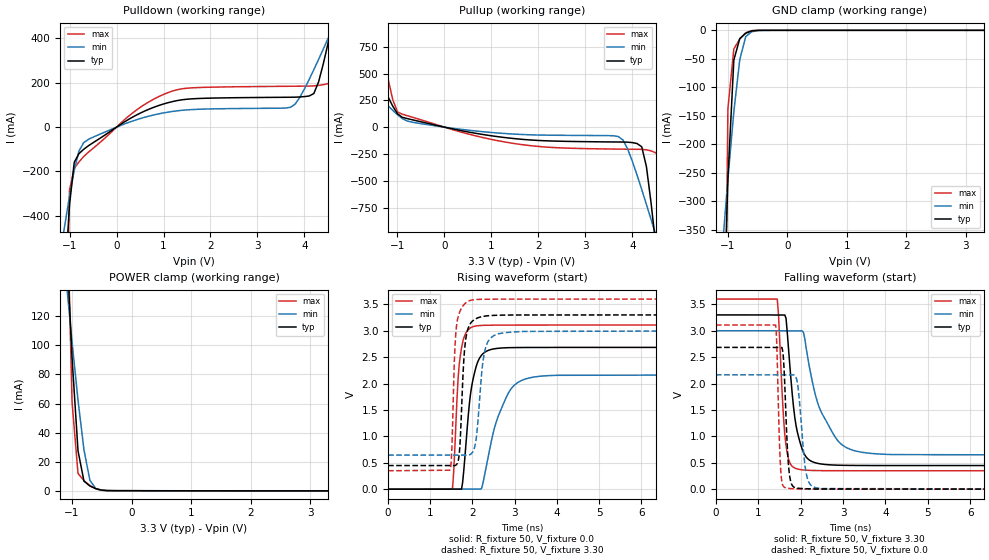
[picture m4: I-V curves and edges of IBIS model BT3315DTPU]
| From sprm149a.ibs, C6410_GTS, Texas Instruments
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[Model]   BT3315DTPU
Model_type   I/O
Vinh = 2.00
Vinl = 0.80
Enable   Active-Low
Polarity   Non-Inverting
| signals   A, GZ, Y
Vmeas = 1.5
|   typ   min   max
C_comp   1.6130p   1.5354p   1.7989p
|   typ   min   max
[Temperature Range]   25   -40   125
|   typ   min   max
[Voltage Range]   3.30V   3.00V   3.60V
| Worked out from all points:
|   slope of the pulldown table from 0 to 0.495 V, typ, clamps not added: 7.97 ohm
|   slope of the pullup table from 0 to 0.495 V, typ, clamps not added: 11.2 ohm
|   GND clamp passes 1 mA (typ) near -0.60 V on its own axis
|   POWER clamp passes 1 mA (typ) near -0.56 V on its own axis
|   rising waveform, R_fixture 50, V_fixture 0.0: 20-80 % time 219ps typ, 469ps min, 133ps max; typ from 0 V to 2.69 V
|   falling waveform, R_fixture 50, V_fixture 3.30: 20-80 % time 235ps typ, 561ps min, 133ps max; typ from 3.3 V to 0.447 V
|   rising waveform, R_fixture 50, V_fixture 3.30: 20-80 % time 109ps typ, 160ps min, 84.2ps max; typ from 0.447 V to 3.3 V
|   falling waveform, R_fixture 50, V_fixture 0.0: 20-80 % time 89.3ps typ, 141ps min, 67.2ps max; typ from 2.69 V to 0 V
[Pulldown]
|   Voltage   I(typ)   I(min)   I(max)
-3.3V     -10.57A    -3.704A    -44.33A
-1.1V     -692.7mA   -440.2mA   -1.224A
-1V       -348.9mA   -310.5mA   -283mA
-900mV    -158.9mA   -194.3mA   -185.9mA
-700mV    -100.1mA   -70.14mA   -132.7mA
1V        104.5mA    64.15mA    147.5mA
3.7V      134.9mA    89.32mA    184.4mA
4.2V      151.5mA    259.2mA    186.2mA
4.6V      471.8mA    446.1mA    223mA
4.7V      570.7mA    493.9mA    367.4mA
4.8V      671.3mA    542mA      570.8mA
6.6V      2.552A     1.425A     4.922A
[GND_clamp]
|   Voltage   I(typ)   I(min)   I(max)
-3.3V     -10.46A    -3.63A     -44.21A
-1.1V     -613.5mA   -391.3mA   -1.123A
-1V       -261.1mA   -261.1mA   -137.8mA
-900mV    -52.05mA   -142.6mA   -32.57mA
-800mV    -14.47mA   -51.16mA   -15.18mA
-700mV    -5.111mA   -10.97mA   -4.271mA
-600mV    -965.9uA   -2.449mA   -468.2uA
-400mV    -4.855uA   -52.49uA   -479.3nA
3.3V      88.82pA    4.205uA    44.41pA
[Pullup]
|   Voltage   I(typ)   I(min)   I(max)
-3.3V     2.442A     1.205A     5.525A
-2.7V     1.813A     912.6mA    4.046A
-1.9V     980.9mA    525.9mA    2.088A
-1.5V     573.5mA    336.5mA    1.13A
-1.1V     195.3mA    156.4mA    256.1mA
-800mV    80.54mA    58.25mA    108mA
3.7V      -138.7mA   -87.82mA   -205mA
4.2V      -183.2mA   -582.4mA   -207.6mA
4.5V      -1.109A    -1.007A    -239.2mA
4.6V      -1.528A    -1.151A    -325.8mA
4.7V      -1.958A    -1.297A    -1.261A
6.6V      -10.56A    -4.136A    -38.31A
[POWER_clamp]
|   Voltage   I(typ)   I(min)   I(max)
-3.3V     2.438A     1.199A     5.524A
-1.1V     176.6mA    145.4mA    226.9mA
-1V       91.69mA    102.4mA    60.94mA
-900mV    27.5mA     62.33mA    11.91mA
-800mV    6.572mA    28.18mA    6.905mA
-700mV    3.22mA     7.14mA     3.606mA
-600mV    1.379mA    1.452mA    1.304mA
-500mV    357.9uA    341.4uA    241uA
-400mV    65.66uA    67.61uA    56.94uA
3.3V      -108.4uA   -68.37uA   -162.2uA
[Ramp]
|   I(typ)   I(min)   I(max)
dV/dt_r   1.611/0.219n   1.299/0.468n   1.865/0.132n
dV/dt_f   1.712/0.234n   1.413/0.562n   1.951/0.132n
[Rising Waveform]
R_fixture = 50
V_fixture = 0.0
|  pu_on
|  TIME   V(typ)   V(min)   V(max)
0s        1nV        11nV       1nV
1.528ns   914.9uV    161.8uV    30.73mV
1.687ns   914.9uV    477uV      2.368V
1.767ns   128.7mV    922uV      2.78V
2.006ns   2.051V     937.6uV    3.075V
2.218ns   2.539V     16.95mV    3.101V
2.536ns   2.66V      1.201V     3.106V
2.801ns   2.678V     1.739V     3.107V
3.252ns   2.683V     2.086V     3.108V
10ns      2.685V     2.165V     3.108V
[Falling Waveform]
R_fixture = 50
V_fixture = 3.30
V_fixture_min = 3.00
V_fixture_max = 3.60
|  pd_on
|  TIME   V(typ)   V(min)   V(max)
0s        3.3V       3V         3.6V
1.446ns   3.298V     3V         3.6V
1.624ns   3.298V     2.998V     1.04V
1.712ns   2.658V     2.998V     570.9mV
1.89ns    1.204V     2.998V     390.8mV
2.067ns   693.5mV    2.961V     363.4mV
2.303ns   510.9mV    1.929V     353.6mV
2.481ns   477.1mV    1.468V     351.3mV
3.19ns    449.9mV    748.9mV    349mV
10ns      447mV      645mV      348.6mV
[Rising Waveform]
R_fixture = 50
V_fixture = 3.30
V_fixture_min = 3.00
V_fixture_max = 3.60
|  pd_off
|  TIME   V(typ)   V(min)   V(max)
0s        447mV      644.9mV    348.6mV
1.458ns   447mV      645.3mV    358.8mV
1.625ns   468.1mV    645.4mV    3.111V
1.699ns   787.8mV    645.4mV    3.357V
1.811ns   2.623V     645.4mV    3.506V
1.922ns   3.095V     648.4mV    3.566V
2.089ns   3.23V      958.1mV    3.591V
2.293ns   3.277V     2.623V     3.596V
2.571ns   3.293V     2.933V     3.598V
10ns      3.3V       3V         3.6V
[Falling Waveform]
R_fixture = 50
V_fixture = 0.0
|  pu_off
|  TIME   V(typ)   V(min)   V(max)
0s        2.685V     2.165V     3.108V
1.408ns   2.684V     2.165V     3.107V
1.529ns   2.684V     2.164V     347.1mV
1.636ns   1.729V     2.164V     27.53mV
1.703ns   546.6mV    2.164V     15.58mV
1.769ns   129mV      2.164V     10.57mV
1.93ns    17.48mV    1.972V     5.213mV
2.144ns   7.92mV     247mV      2.361mV
2.331ns   4.54mV     32.68mV    1.392mV
10ns      260.4nV    3.865uV    131nV
